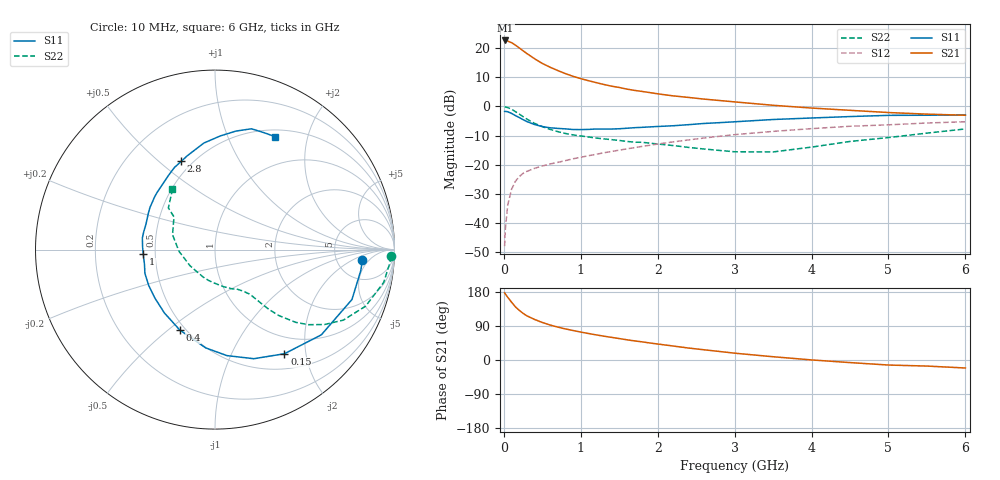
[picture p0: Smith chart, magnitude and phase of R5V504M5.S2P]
! SIEMENS Small Signal Semiconductors
! BFR183
! Si NPN RF Bipolar Junction Transistor in SOT23
! VCE = 0.5 V  IC = 4.5 mA
! Common Emitter S-Parameters:  May  1996
# GHz  S  MA  R  50
!  f  S11  S21  S12  S22
! GHz  MAG  ANG  MAG  ANG  MAG  ANG  MAG  ANG
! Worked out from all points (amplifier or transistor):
!   36 points, 10 MHz to 6 GHz, reference 50 ohm
!   highest |S21| = 22.6 dB at 20 MHz (marker M1)
!   |S21| within 3 dB of that: start of sweep to 222.5 MHz
!   unconditionally stable (mu >= 1): 945.9 MHz to 3.475 GHz
!   at 250 MHz: K = 0.41, MSG = 21.0 dB, |S12| = -23.0 dB
!   at 1.4 GHz: K = 1.10, MAG = 9.2 dB, |S12| = -15.4 dB
!   at 6 GHz: K = 0.98, MSG = 1.1 dB, |S12| = -5.3 dB
!   S11 on the Smith chart (normalised r, x): 10 MHz: 9.08, -3.31; 150 MHz: 0.72, -1.63; 400 MHz: 0.47, -0.55; 1 GHz: 0.43, -0.03; 2.8 GHz: 0.44, +0.60; 6 GHz: 0.59, +1.51
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0.01  0.8231 -4.1  13.42 177.3  0.004 87.8  0.9821 -2.2
0.02  0.8206 -8.2  13.57 174.0  0.008 83.0  0.9766 -4.5
0.05  0.8122 -20.0  13.24 165.6  0.0201 79.4  0.9577 -11.0
0.1  0.7593 -38.7  12.43 152.6  0.0378 71.0  0.8962 -20.6
0.15  0.6974 -56.3  11.3 140.2  0.0518 62.7  0.8158 -28.8
0.2  0.6453 -70.4  10.11 131.2  0.0625 57.5  0.7389 -34.4
0.25  0.5943 -83.6  9.02 123.1  0.071 53.7  0.6677 -38.8
0.3  0.5501 -95.4  8.085 116.5  0.0769 51.4  0.6059 -42.0
0.4  0.4889 -113.7  6.584 107.0  0.0868 48.3  0.5123 -45.9
0.5  0.4518 -128.6  5.472 99.0  0.095 47.1  0.4505 -47.9
0.6  0.4303 -141.1  4.723 92.4  0.1029 46.9  0.4048 -49.1
0.8  0.4123 -161.3  3.661 82.0  0.1176 47.8  0.3437 -50.9
1  0.4007 -176.4  3.001 73.7  0.1342 48.4  0.3117 -52.3
1.1  0.4037 177.8  2.767 69.9  0.1426 48.9  0.2992 -53.7
1.3  0.4093 165.7  2.382 62.9  0.1601 49.1  0.2774 -56.0
1.6  0.4227 151.5  1.983 53.3  0.1872 49.0  0.2509 -61.1
2.2  0.466 129.0  1.519 36.9  0.2466 45.9  0.2133 -76.4
2.8  0.5265 110.9  1.265 22.6  0.3069 40.3  0.1759 -101.3
3.5  0.5968 96.0  1.047 8.6  0.3731 31.7  0.1657 -146.9
4.5  0.6705 80.0  0.858 -6.8  0.4569 18.9  0.2508 160.7
5.5  0.7064 67.2  0.738 -16.0  0.5197 7.4  0.3485 138.2
6  0.7131 61.8  0.706 -21.1  0.546 -0.2  0.4111 125.2
